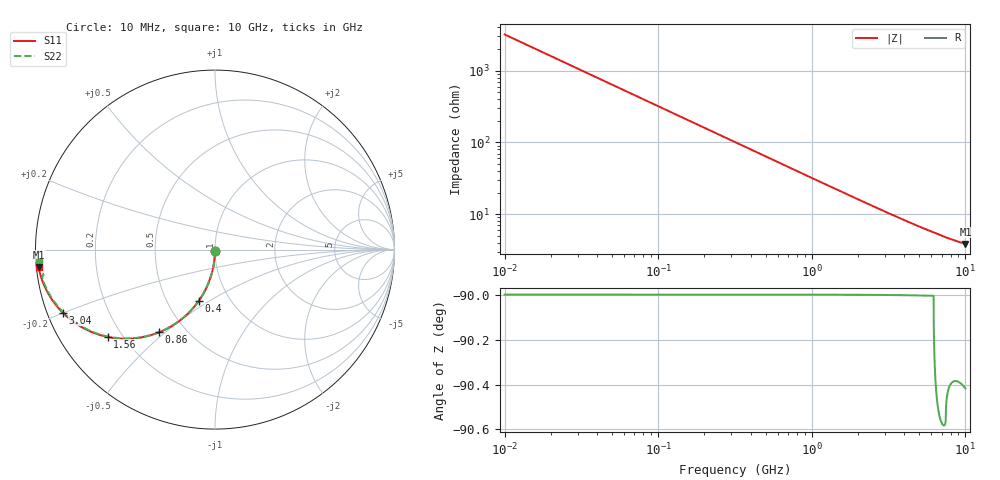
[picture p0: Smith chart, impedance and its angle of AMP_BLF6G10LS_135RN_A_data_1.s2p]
! Created Thu Oct 22 13:03:40 2009
# ghz S ma R 50
! 2 Port Network Data from SP1.SP block
! freq  magS11  angS11  magS21  angS21  magS12  angS12  magS22  angS22
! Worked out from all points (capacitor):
!   1000 points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, 10 MHz to 10 GHz, reference 50 ohm
!   read as one part in shunt: C = 4.99 pF near 60 MHz
!   lowest |Z| = 3.86 ohm at 10 GHz (marker M1)
!   S11 on the Smith chart (normalised r, x): 10 MHz: 1.00, -0.02; 400 MHz: 0.72, -0.45; 860 MHz: 0.36, -0.48; 1.56 GHz: 0.15, -0.35; 3.04 GHz: 0.04, -0.20; 10 GHz: 0.01, -0.05
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0.01  0.007807 -90.4  1 -0.5  1 -0.5  0.007807 -90.4
0.03  0.02342 -91.3  0.9997 -1.4  0.9997 -1.4  0.02342 -91.4
0.07  0.05457 -93.1  0.9985 -3.2  0.9985 -3.2  0.05457 -93.2
0.08  0.06233 -93.6  0.9981 -3.6  0.9981 -3.6  0.06233 -93.6
0.1  0.07783 -94.5  0.997 -4.5  0.997 -4.5  0.07783 -94.5
0.13  0.101 -95.8  0.9949 -5.8  0.9949 -5.8  0.101 -95.9
0.18  0.1391 -98.0  0.9903 -8.1  0.9903 -8.1  0.1391 -98.1
0.24  0.1841 -100.7  0.9829 -10.7  0.9829 -10.7  0.1841 -100.7
0.31  0.2351 -103.7  0.972 -13.7  0.972 -13.7  0.2351 -103.7
0.4  0.2979 -107.4  0.9546 -17.5  0.9546 -17.5  0.2979 -107.5
0.6  0.4237 -115.2  0.9058 -25.3  0.9058 -25.3  0.4237 -115.3
0.86  0.5564 -124.0  0.8309 -34.1  0.8309 -34.1  0.5564 -124.2
1.17  0.6728 -132.6  0.7398 -42.7  0.7398 -42.7  0.6728 -132.8
1.56  0.7706 -140.8  0.6373 -51.0  0.6373 -51.0  0.7706 -141.1
1.68  0.7928 -142.9  0.6095 -53.1  0.6095 -53.1  0.7928 -143.2
2.28  0.8689 -151.0  0.495 -61.2  0.495 -61.2  0.8689 -151.4
3.04  0.9183 -157.5  0.3959 -67.8  0.3959 -67.8  0.9183 -158.1
3.34  0.9304 -159.4  0.3665 -69.7  0.3665 -69.7  0.9304 -160.1
5.01  0.9653 -166.3  0.2609 -76.8  0.2609 -76.8  0.9653 -167.4
6.67  0.9782 -170.0  0.2053 -81.4  0.2053 -81.4  0.9664 -171.6
8.34  0.9848 -172.5  0.1722 -83.6  0.1722 -83.6  0.9776 -173.9
10  0.988 -174.3  0.1525 -85.6  0.1525 -85.6  0.9815 -176.0
